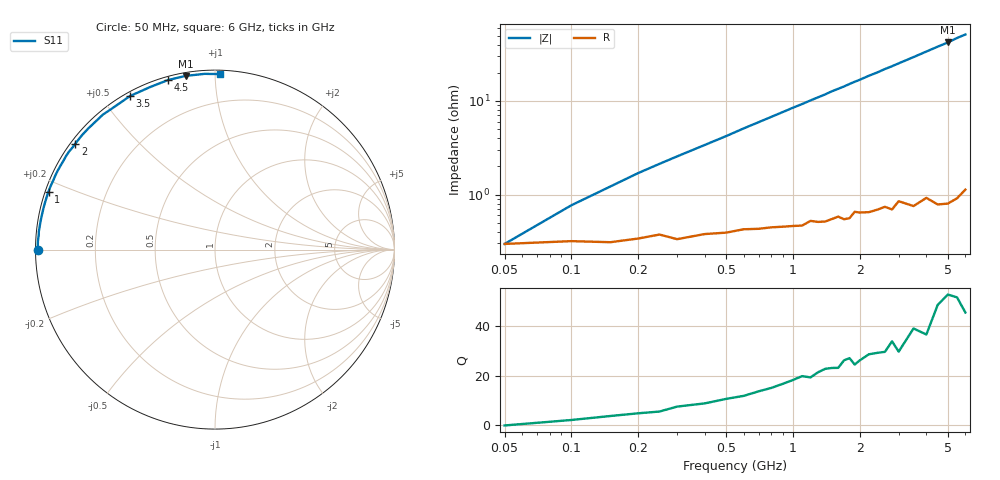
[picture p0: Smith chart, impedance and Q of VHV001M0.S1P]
! Infineon Technologies  Discrete & RF Semiconductors
! BB 814
! Si Tuning Diode in SOT23
! VR =
! S-Parameters:  July  1999
# GHz  S  MA  R  50
!  f  S11
! GHz  MAG  ANG
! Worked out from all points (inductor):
!   34 points, 50 MHz to 6 GHz, reference 50 ohm
!   read as one part to ground: L = 1.32 nH near 150 MHz
!   highest Q = 51.7 at 5 GHz (marker M1), where L = 1.34 nH
!   S11 on the Smith chart (normalised r, x): 50 MHz: 0.01, +0.00; 1 GHz: 0.01, +0.17; 2 GHz: 0.01, +0.34; 3.5 GHz: 0.02, +0.59; 4.5 GHz: 0.02, +0.76; 6 GHz: 0.02, +1.03
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0.05  0.9882 180.0
0.1  0.9874 178.4
0.2  0.9866 176.2
0.25  0.9852 175.2
0.3  0.9868 174.2
0.5  0.9846 170.4
0.6  0.9833 168.4
0.8  0.9826 164.6
1  0.9822 160.8
1.1  0.9822 159.0
1.4  0.9807 153.5
1.5  0.9797 151.5
1.6  0.9786 149.8
1.7  0.9801 148.1
1.8  0.9797 146.2
1.9  0.9766 144.4
2  0.9772 142.8
2.2  0.9775 139.2
2.4  0.9766 136.1
2.6  0.9755 132.6
2.8  0.9776 129.6
3  0.9733 126.4
3.5  0.9779 119.0
4  0.975 111.9
4.5  0.9804 105.4
5  0.9815 99.6
5.5  0.9809 93.4
6  0.9783 88.4
